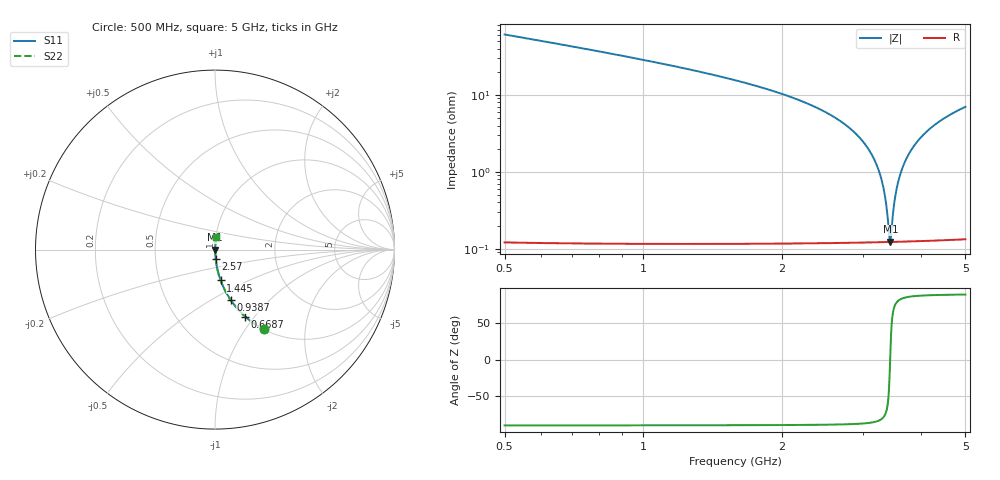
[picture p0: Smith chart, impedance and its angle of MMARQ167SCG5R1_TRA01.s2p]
! MMARQ167SCG5R1_TRA01  S-PARAMETER MODEL  ( General Type )
! Model Generated by TAIYO YUDEN Corporation (http://www.ty-top.com)
! Version 1.0
! TAIYO YUDEN Control No. 160201
! Copyright(c) 2016 TAIYO YUDEN CO.,LTD. All Rights Reserved.
! Product Description (link to TY-COMPAS)
! https://ds.yuden.co.jp/TYCOMPAS/or/detail?pn=MMARQ167SCG5R1CTRA01&u=M
! Products Name : Multilayer Ceramic Capacitors
! Characteristics :
!  Capacitance : 5.1 pF , Rated Voltage : 250V , TCC : CG / C0G
!  Case Size : 1.6 x 0.8 / 0.063 x 0.031 [mm/inch] , Thickness : 0.7 / 0.028 [mm/inch]
!  (Conditions: Temperature = 25 degC , DC Bias Current/Voltage = 0A / 0V)
! External Node Assignments :
!  1  o---| |---o  2
! GND o---------o GND
! Frequency Range : 500MHz  -  5000MHz  [ 401 STEP ]
# MHz S RI R 50
! Freq[MHz].  S11 Real  S11 Imag  S21 Real  S21 Imag  S12 Real  S12 Imag  S22 Real  S22 Imag
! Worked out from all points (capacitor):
!   401 points, 500 MHz to 5 GHz, reference 50 ohm
!   read as one part in series: C = 5.1 pF near 522.5 MHz
!   lowest |Z| = 124 mohm at 3.436 GHz (marker M1)
!   series resonance near 3.433 GHz, so ESL is about 420 pH
!   S11 on the Smith chart (normalised r, x): 500 MHz: 1.00, -1.22; 668.8 MHz: 1.00, -0.90; 938.8 MHz: 1.00, -0.61; 1.445 GHz: 1.00, -0.36; 2.57 GHz: 1.00, -0.11; 5 GHz: 1.00, +0.14
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500  0.272 -0.444  0.728 0.444  0.728 0.444  0.272 -0.444
668.75  0.1683 -0.3728  0.8317 0.3728  0.8317 0.3728  0.1683 -0.3728
938.75  0.0872 -0.2803  0.9128 0.2803  0.9128 0.2803  0.0872 -0.2803
1253.75  0.0454 -0.2056  0.9546 0.2056  0.9546 0.2056  0.0454 -0.2056
1445  0.0316 -0.1718  0.9684 0.1718  0.9684 0.1718  0.0316 -0.1718
2007.5  0.0115 -0.101  0.9885 0.101  0.9885 0.101  0.0115 -0.101
2570  0.00401 -0.0531  0.996 0.0531  0.996 0.0531  0.00401 -0.0531
2750  0.00283 -0.0405  0.9972 0.0405  0.9972 0.0405  0.00283 -0.0405
3031.25  0.00172 -0.0226  0.9983 0.0226  0.9983 0.0226  0.00172 -0.0226
3222.5  0.00134 -0.0115  0.9987 0.0115  0.9987 0.0115  0.00134 -0.0115
3335  0.00125 -0.00524  0.9988 0.00524  0.9988 0.00524  0.00125 -0.00524
3368.75  0.00123 -0.00341  0.9988 0.00341  0.9988 0.00341  0.00123 -0.00341
3413.75  0.00122 -0.00101  0.9988 0.00101  0.9988 0.00101  0.00122 -0.00101
3436.25  0.00122 0.000185  0.9988 -0.000185  0.9988 -0.000185  0.00122 0.000185
3458.75  0.00123 0.00137  0.9988 -0.00137  0.9988 -0.00137  0.00123 0.00137
3503.75  0.00124 0.00371  0.9988 -0.00371  0.9988 -0.00371  0.00124 0.00371
3548.75  0.00127 0.00603  0.9987 -0.00603  0.9987 -0.00603  0.00127 0.00603
3593.75  0.0013 0.00831  0.9987 -0.00831  0.9987 -0.00831  0.0013 0.00831
3740  0.00148 0.0156  0.9985 -0.0156  0.9985 -0.0156  0.00148 0.0156
3953.75  0.00191 0.0257  0.9981 -0.0257  0.9981 -0.0257  0.00191 0.0257
4257.5  0.00282 0.0393  0.9972 -0.0393  0.9972 -0.0393  0.00282 0.0393
5000  0.00618 0.0695  0.9938 -0.0695  0.9938 -0.0695  0.00618 0.0695
